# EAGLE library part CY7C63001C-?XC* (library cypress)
Universal Serial Bus Microcontroller Integrated USB transceiver Source: www.cypress.com .. CY7C6301XX.pdf
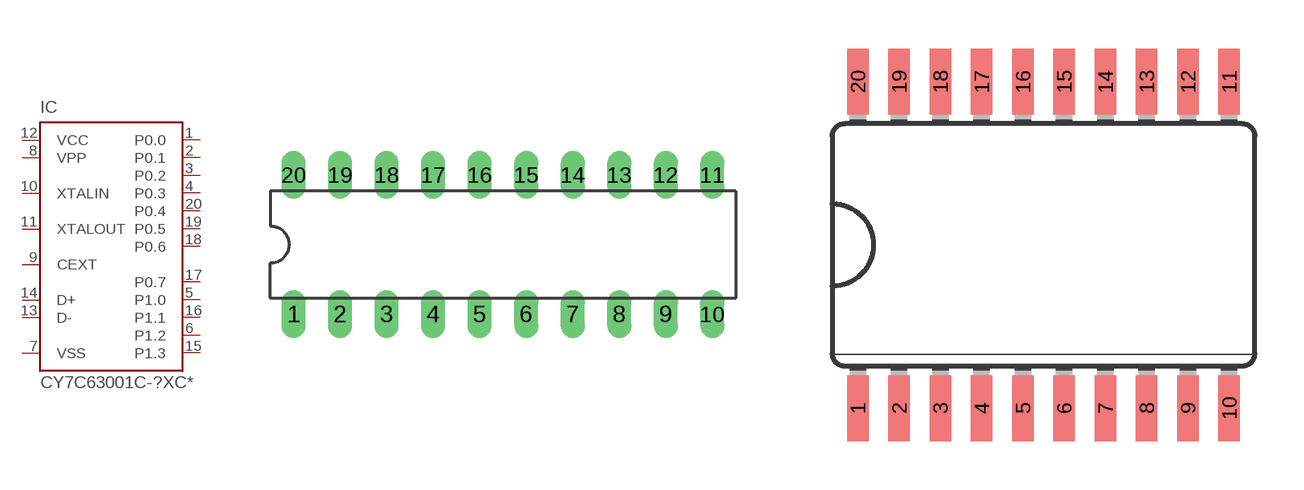
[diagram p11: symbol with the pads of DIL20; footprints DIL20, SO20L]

Designator prefix IC

## CY7C63001C-PXC (MPN: CY7C63001C-PXC; OC_FARNELL: unknown; OC_NEWARK: 19M7032)  [DIL20]
1  P0.0
2  P0.1
3  P0.2
4  P0.3
5  P1.0
6  P1.2
7  VSS  pwr
8  VPP  in
9  CEXT  pas
10  XTALIN  in
11  XTALOUT  out
12  VCC  pwr
13  D-
14  D+
15  P1.3
16  P1.1
17  P0.7
18  P0.6
19  P0.5
20  P0.4

## CY7C63001C-SXC (MPN: CY7C63001C-SXC; OC_FARNELL: 1769872; OC_NEWARK: 19M7033), CY7C63001C-SXCT (MPN: CY7C63001C-SXCT; OC_FARNELL: unknown; OC_NEWARK: 19M7034)  [SO20L]
Pads as for DIL20

## Footprint DIL20 (pad centres in mm)
Dual In Line Package
drill 0.813 long: 1 -11.43,-3.81; 2 -8.89,-3.81; 3 -6.35,-3.81; 4 -3.81,-3.81; 5 -1.27,-3.81; 6 1.27,-3.81; 7 3.81,-3.81; 8 6.35,-3.81; 9 8.89,-3.81; 10 11.43,-3.81; 11 11.43,3.81; 12 8.89,3.81; 13 6.35,3.81; 14 3.81,3.81; 15 1.27,3.81; 16 -1.27,3.81; 17 -3.81,3.81; 18 -6.35,3.81; 19 -8.89,3.81; 20 -11.43,3.81

## Footprint SO20L (pad centres in mm)
20-Lead (300-MIL) SOIC S5 Source: www.cypress.com .. CY7C6301XX.pdf
smd 0.66 x 2.032: 1 -5.715,-5.029; 2 -4.445,-5.029; 3 -3.175,-5.029; 4 -1.905,-5.029; 5 -0.635,-5.029; 6 0.635,-5.029; 7 1.905,-5.029; 8 3.175,-5.029; 9 4.445,-5.029; 10 5.715,-5.029; 11 5.715,5.029; 12 4.445,5.029; 13 3.175,5.029; 14 1.905,5.029; 15 0.635,5.029; 16 -0.635,5.029; 17 -1.905,5.029; 18 -3.175,5.029; 19 -4.445,5.029; 20 -5.715,5.029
